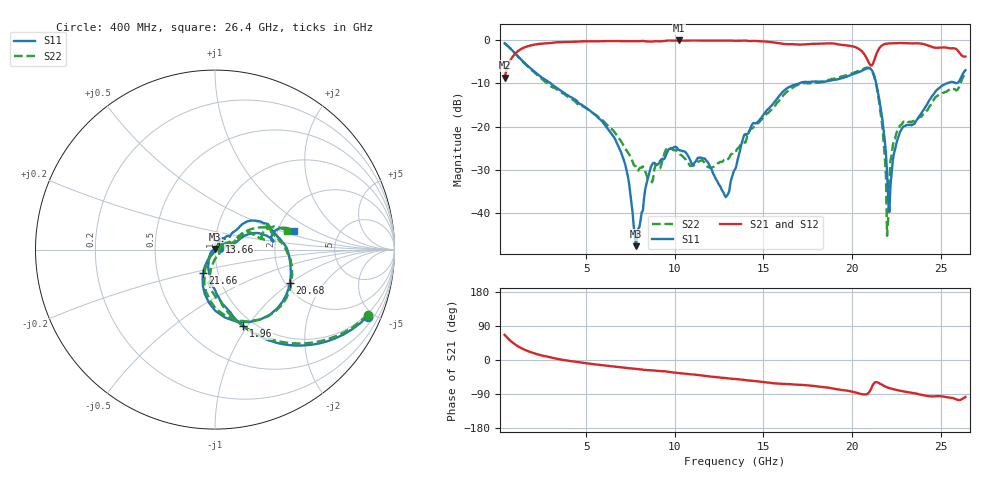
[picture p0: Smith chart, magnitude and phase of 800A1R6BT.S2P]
!  American Technical Ceramics  Date:  12/17/08
!  One Norden Lane
!  Huntington Station,  NY.  11746-2102
!  Tel:  (631) 622-4700  Fax:  (631) 622-4748
!  Part Number  800A1R6BT
!  Description: Broardband capacitor  Mounting Orientation: Vertical
!  Application:
# GHZ S DB R 50
! Freq  |S11|  S11 Ph  |S21|  S21 Ph  |S12|  S12 Ph  |S22|  S22 Ph
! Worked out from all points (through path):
!   401 points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, 400 MHz to 26.4 GHz, reference 50 ohm
!   highest |S21| = 0.00 dB at 10.21 GHz (marker M1); lowest = -8.6 dB at 400 MHz (marker M2)
!   group delay of S21, straight-line fit = 13.5 ps
!   lowest |S11| = -47.8 dB at 7.81 GHz (marker M3), VSWR 1.01, Z = 49.8 + j0.329 ohm
!   |S11| at or under -10 dB: 3.012 GHz to 17.01 GHz (14 GHz wide, 140 % of centre); 21.37 GHz to 25.33 GHz (3.967 GHz wide, 17 % of centre)
!   |S22| runs from -45.4 to -0.7 dB; largest |S21 - S12| = 0.0086
!   S11 on the Smith chart (normalised r, x): 400 MHz: 0.86, -4.61; 1.96 GHz: 0.89, -0.96; 13.66 GHz: 1.04, +0.09; 20.68 GHz: 2.12, -1.00; 21.66 GHz: 0.85, -0.23; 26.4 GHz: 2.44, +0.64
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0.4  -0.65 -23.7  -8.61 66.4  -8.65 66.4  -0.68 -23.0
1.96  -6.83 -69.6  -1.07 19.3  -1.10 19.4  -7.01 -70.4
4.755  -14.96 -96.2  -0.21 -7.1  -0.23 -6.9  -15.18 -99.0
6.9  -25.36 -127.2  -0.14 -19.1  -0.14 -18.8  -23.02 -97.1
7.81  -47.80 125.7  -0.16 -23.5  -0.14 -23.2  -29.28 -64.1
8.59  -30.39 55.7  -0.26 -27.1  -0.24 -26.7  -32.49 -15.6
9.11  -28.57 38.0  -0.21 -29.0  -0.19 -28.6  -29.60 18.1
10.215  -25.39 11.3  0.00 -34.7  -0.01 -34.4  -26.12 21.6
11.775  -27.89 -14.2  -0.01 -42.4  -0.01 -42.3  -29.02 35.8
12.88  -36.42 14.0  -0.01 -47.8  -0.01 -47.7  -28.02 29.2
13.4  -29.98 57.3  -0.08 -50.1  -0.06 -50.1  -25.67 23.5
13.66  -25.97 65.0  -0.06 -51.1  -0.04 -51.1  -24.62 22.8
16.13  -11.78 38.8  -0.81 -63.1  -0.78 -63.2  -12.70 29.6
17.755  -9.54 20.4  -0.79 -68.2  -0.76 -68.3  -9.88 22.7
20.68  -6.79 -24.0  -3.12 -91.0  -3.08 -91.2  -6.53 -26.6
21.2  -7.56 -73.4  -5.25 -64.0  -5.22 -64.3  -7.70 -73.0
21.655  -16.69 -116.9  -1.27 -64.3  -1.24 -64.7  -18.08 -116.9
21.915  -26.18 -124.4  -0.77 -70.8  -0.74 -71.2  -31.31 -119.7
22.11  -39.82 -34.3  -0.68 -74.2  -0.65 -74.5  -32.49 28.5
22.305  -27.86 11.1  -0.65 -76.7  -0.62 -77.1  -24.44 29.9
22.695  -21.44 13.5  -0.60 -80.9  -0.57 -81.4  -19.83 23.9
26.4  -6.93 13.5  -3.73 -97.7  -3.70 -98.2  -7.63 14.5
